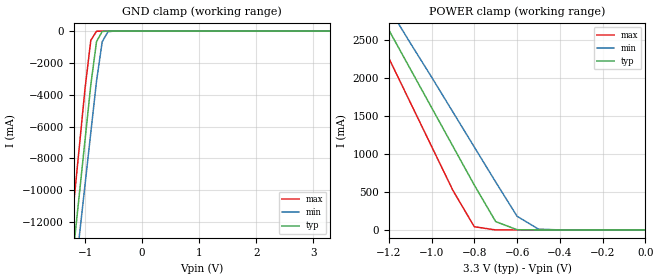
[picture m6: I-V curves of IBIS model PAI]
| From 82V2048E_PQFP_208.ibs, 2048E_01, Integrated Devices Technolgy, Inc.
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|   Model PAI
[Model]   PAI
Model_type   Input
Polarity   Non-Inverting
Vinl =   0.74V
Vinh =   2.10V
C_comp   3.50pF   4.00pF   3.50pF
[Temperature Range]   25.00   85.00   -40.00
[Voltage Range]   3.30V   3.00V   3.60V
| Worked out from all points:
|   GND clamp passes 1 mA (typ) near -0.60 V on its own axis
|   POWER clamp passes 1 mA (typ) near -0.53 V on its own axis
[GND_clamp]
| voltage   I(typ)   I(min)   I(max)
-3.3V     -85.43A    -84.06A    -87.29A
-1.3V     -17.05A    -19.32A    -14.49A
-1.2V     -13.63A    -16.08A    -10.85A
-1.1V     -10.21A    -12.85A    -7.21A
-1V       -6.8A      -9.61A     -3.57A
-900mV    -3.38A     -6.37A     -580mA
-800mV    -660mA     -3.14A     -10.67mA
-700mV    -22.9mA    -670mA     -690uA
-600mV    -510uA     -40.64mA   -38.38uA
-400mV    -350nA     -64.42uA   -25.6nA
3.3V      3.48pA     17.52uA    3pA
[POWER_clamp]
| voltage   I(typ)   I(min)   I(max)
-3.3V     13.35A     12.56A     14.47A
-1.3V     3.14A      3.38A      2.84A
-1.2V     2.63A      2.92A      2.26A
-1.1V     2.12A      2.46A      1.68A
-900mV    1.1A       1.55A      520mA
-800mV    590mA      1.09A      42.64mA
-700mV    110mA      630mA      350uA
-600mV    3.23mA     180mA      2.46uA
-500mV    66.65uA    11.08mA    17.16nA
-400mV    1.36uA     450uA      120pA
0V        3.48pA     160pA      3.6pA
